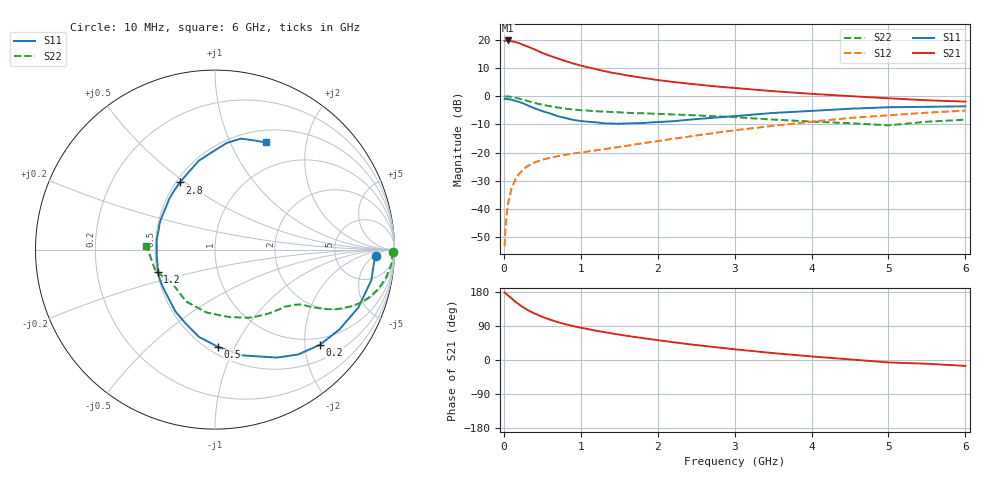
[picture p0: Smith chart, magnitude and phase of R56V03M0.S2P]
! SIEMENS Small Signal Semiconductors
! BFR183
! Si NPN RF Bipolar Junction Transistor in SOT23
! VCE = 6 V  IC = 3 mA
! Common Emitter S-Parameters:  May  1996
# GHz  S  MA  R  50
!  f  S11  S21  S12  S22
! GHz  MAG  ANG  MAG  ANG  MAG  ANG  MAG  ANG
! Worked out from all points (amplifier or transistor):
!   36 points, 10 MHz to 6 GHz, reference 50 ohm
!   highest |S21| = 19.7 dB at 50 MHz (marker M1)
!   |S21| within 3 dB of that: start of sweep to 385 MHz
!   unconditionally stable (mu >= 1): 1.27 GHz to 2.795 GHz
!   at 250 MHz: K = 0.29, MSG = 22.1 dB, |S12| = -26.0 dB
!   at 1.4 GHz: K = 1.04, MAG = 12.1 dB, |S12| = -18.4 dB
!   at 6 GHz: K = 0.89, MSG = 1.6 dB, |S12| = -5.1 dB
!   lowest NFmin = 1.10 dB at 450 MHz
!   S11 on the Smith chart (normalised r, x): 10 MHz: 16, -6; 200 MHz: 0.83, -2.34; 500 MHz: 0.56, -0.86; 1.2 GHz: 0.50, -0.14; 2.8 GHz: 0.52, +0.48; 6 GHz: 0.65, +1.37
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0.01  0.895 -2.3  9.502 178.4  0.0022 86.1  0.9942 -0.9
0.02  0.8888 -4.7  9.608 176.2  0.0046 84.6  0.9878 -1.9
0.05  0.8876 -11.1  9.673 171.1  0.0118 83.9  0.9865 -4.8
0.1  0.8615 -21.9  9.326 162.7  0.0233 78.2  0.9659 -9.3
0.15  0.8239 -32.7  9.079 153.5  0.0335 72.4  0.9367 -13.5
0.2  0.7891 -42.2  8.634 146.3  0.0424 67.9  0.9018 -17.0
0.3  0.6935 -60.2  7.627 132.8  0.0568 60.9  0.828 -22.3
0.4  0.6084 -75.6  6.719 122.6  0.0669 55.7  0.7574 -26.0
0.5  0.5419 -88.3  5.798 113.7  0.0747 52.4  0.7023 -28.2
0.6  0.4948 -100.3  5.163 106.5  0.0809 50.3  0.6618 -29.5
0.7  0.441 -112.2  4.646 100.1  0.0862 49.7  0.6286 -30.6
0.8  0.4093 -122.6  4.175 94.4  0.0912 48.9  0.6 -31.5
0.9  0.3797 -131.7  3.792 89.5  0.0961 49.6  0.5777 -32.1
1.1  0.3511 -150.1  3.218 81.3  0.105 50.1  0.5515 -33.8
1.2  0.3432 -158.5  2.989 77.2  0.1097 50.5  0.5397 -34.7
1.6  0.3286 171.5  2.33 63.7  0.1321 53.3  0.5069 -38.7
2.2  0.3592 140.3  1.783 47.0  0.1755 55.4  0.4738 -47.1
2.8  0.4225 117.6  1.466 32.8  0.2279 53.9  0.4364 -58.9
3.5  0.5033 100.4  1.222 18.2  0.2974 48.4  0.3839 -78.3
4.5  0.5974 83.8  1 1.6  0.4107 37.2  0.3309 -119.2
5.5  0.6461 70.3  0.844 -9.9  0.5086 24.0  0.3522 -160.1
6  0.6606 64.6  0.799 -15.6  0.5534 15.4  0.3825 176.8
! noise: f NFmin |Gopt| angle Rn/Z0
0.45  1.1  0.37  35  0.3
0.9  1.15  0.34  85  0.23
1.8  1.9  0.35  160  0.13
